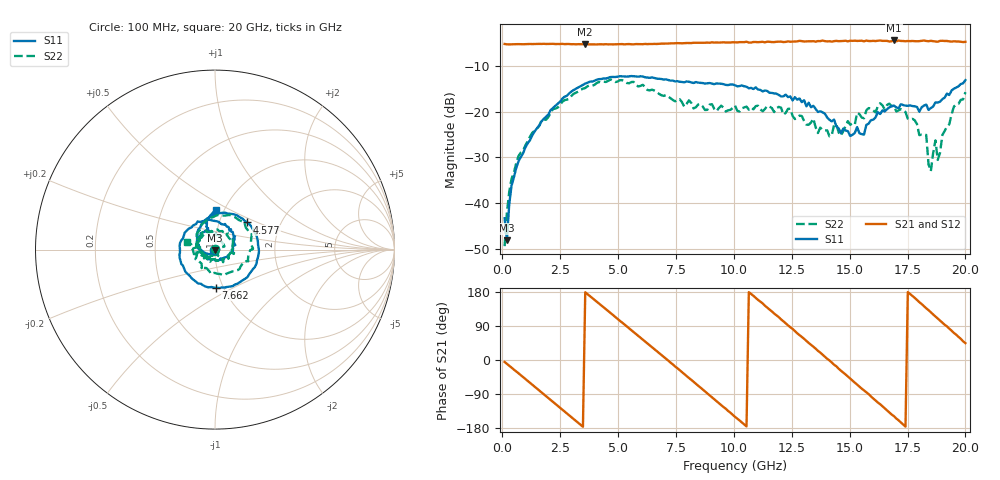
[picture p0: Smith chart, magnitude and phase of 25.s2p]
!Agilent Technologies,N5230C,MY49001569,A.09.33.09
!Agilent N5230C: A.09.33.09
!Date: Sunday, July 26, 2015 10:37:37
!Correction: S11(Full 2 Port(1,2))
!S21(Full 2 Port(1,2))
!S12(Full 2 Port(1,2))
!S22(Full 2 Port(1,2))
!S2P File: Measurements: S11, S21, S12, S22:
# Hz S  dB  R 50
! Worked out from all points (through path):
!   201 points, 100 MHz to 20 GHz, reference 50 ohm
!   highest |S21| = -4.42 dB at 16.92 GHz (marker M1); lowest = -5.3 dB at 3.583 GHz (marker M2)
!   group delay of S21, straight-line fit = 143 ps
!   lowest |S11| = -48.1 dB at 199.5 MHz (marker M3), VSWR 1.01, Z = 50 - j0.392 ohm
!   |S11| at or under -10 dB: start of sweep to end of sweep
!   |S22| runs from -49.4 to -13.0 dB; largest |S21 - S12| = 0.027
!   S11 on the Smith chart (normalised r, x): 100 MHz: 0.99, -0.01; 4.577 GHz: 1.36, +0.43; 7.662 GHz: 0.92, -0.41; 20 GHz: 0.91, +0.42
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1e8  -43.34 -150.0  -5.19 -5.1  -5.25 -5.3  -49.45 78.5
1.995e8  -48.13 -88.8  -5.27 -10.2  -5.27 -10.1  -42.06 -71.9
3.985e8  -36.22 -102.9  -5.26 -19.9  -5.26 -19.9  -34.71 -93.7
6.97e8  -30.91 -123.6  -5.22 -34.8  -5.23 -34.9  -29.75 -113.9
1.9905e9  -20.63 165.9  -5.17 -100.5  -5.17 -100.7  -21.18 175.8
3.483e9  -14.15 90.1  -5.26 -176.2  -5.27 -176.1  -14.99 98.7
3.5825e9  -13.86 84.9  -5.30 178.7  -5.27 178.7  -14.83 93.3
4.5775e9  -12.60 40.2  -5.28 128.9  -5.26 128.8  -13.25 46.5
5.672e9  -12.25 -6.8  -5.27 73.7  -5.22 73.5  -13.48 0.9
6.7665e9  -12.81 -51.7  -5.14 18.4  -5.13 18.3  -16.11 -50.5
7.662e9  -13.46 -88.4  -5.03 -26.8  -5.06 -27.0  -17.27 -100.0
8.856e9  -13.81 -137.6  -4.88 -88.2  -4.86 -88.7  -19.60 -177.2
1.005e10  -14.23 164.1  -4.83 -150.1  -4.85 -150.1  -18.66 115.5
1.204e10  -16.67 76.2  -4.66 107.1  -4.69 106.9  -19.14 6.0
1.3433e10  -18.72 12.6  -4.58 35.2  -4.67 34.1  -21.53 -57.3
1.5224e10  -24.67 -112.1  -4.46 -59.8  -4.44 -59.4  -22.82 -172.8
1.67165e10  -19.08 151.8  -4.65 -138.9  -4.55 -138.9  -18.25 119.0
1.69155e10  -18.69 143.1  -4.42 -148.1  -4.56 -149.5  -18.71 115.5
1.83085e10  -18.46 108.8  -4.53 136.5  -4.50 135.8  -25.09 18.4
1.85075e10  -19.22 110.9  -4.49 125.9  -4.59 125.6  -33.02 -13.0
1.87065e10  -17.97 107.8  -4.63 114.9  -4.61 114.7  -26.29 -54.0
2e10  -13.11 89.1  -4.72 44.5  -4.73 43.8  -15.73 164.7
